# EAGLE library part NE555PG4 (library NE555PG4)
Precision timer, PDIP-8 Source: Datasheet
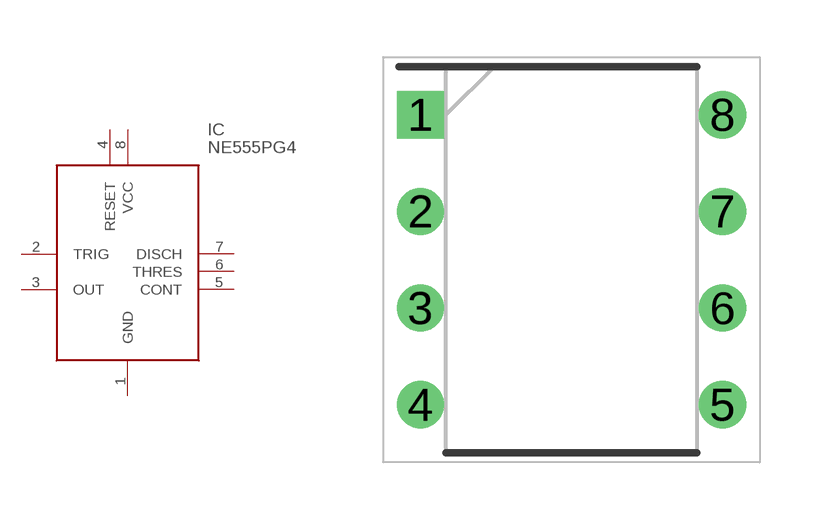
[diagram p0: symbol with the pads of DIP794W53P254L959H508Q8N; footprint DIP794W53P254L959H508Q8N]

Designator prefix IC

## NE555PG4 (Description: Precision timer, PDIP-8; Height: 5.08mm; Manufacturer_Name: Texas Instruments; Manufacturer_Part_Number: NE555PG4)  [DIP794W53P254L959H508Q8N]
1  GND
2  TRIG
3  OUT
4  RESET
5  CONT
6  THRES
7  DISCH
8  VCC

## Footprint DIP794W53P254L959H508Q8N (pad centres in mm)
P (R-PDIP-T8)
drill 0.73 pad 1.13 square: 1 -3.97,3.81
drill 0.73 pad 1.13: 2 -3.97,1.27; 3 -3.97,-1.27; 4 -3.97,-3.81; 5 3.97,-3.81; 6 3.97,-1.27; 7 3.97,1.27; 8 3.97,3.81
